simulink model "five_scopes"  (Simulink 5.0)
settings: Solver=ode45  StartTime=0.0  StopTime=10.0  RelTol=1e-3
libraries: xpclib x5

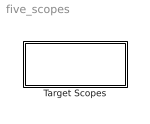
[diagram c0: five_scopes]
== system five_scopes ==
  Target Scopes : Subsystem

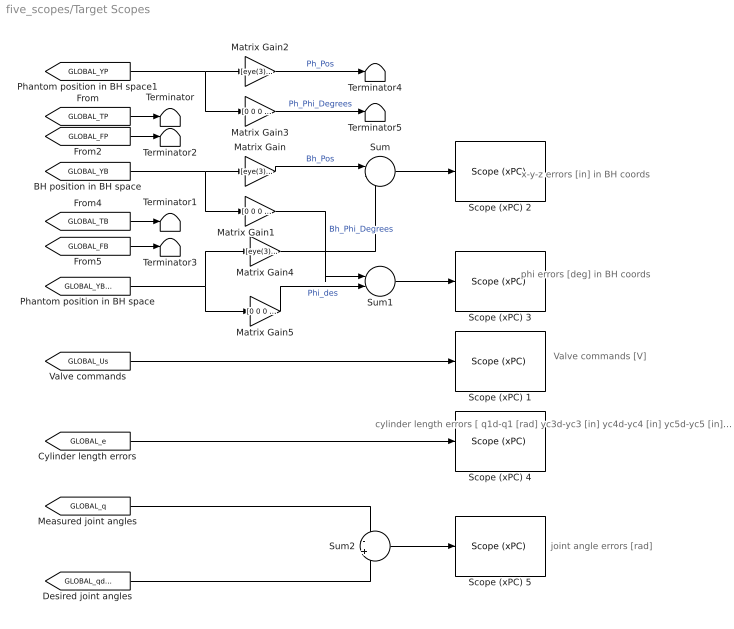
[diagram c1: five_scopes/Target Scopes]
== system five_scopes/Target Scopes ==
  note: x-y-z errors [in] in BH coords
  note: phi errors [deg] in BH coords
  note: Valve commands [V]
  note: cylinder length errors [ q1d-q1 [rad] yc3d-yc3 [in] yc4d-yc4 [in] yc5d-yc5 [in] ]
  note: joint angle errors [rad]
  Matrix Gain : Gain  Gain=[eye(3) zeros(3,1)]  Multiplication=Matrix(K*u)
  Matrix Gain1 : Gain  Gain=[0 0 0 180/pi]  Multiplication=Matrix(K*u)
  Matrix Gain2 : Gain  Gain=[eye(3) zeros(3,1)]  Multiplication=Matrix(K*u)
  Matrix Gain3 : Gain  Gain=[0 0 0 180/pi]  Multiplication=Matrix(K*u)
  Matrix Gain4 : Gain  Gain=[eye(3) zeros(3,1)]  Multiplication=Matrix(K*u)
  Matrix Gain5 : Gain  Gain=[0 0 0 180/pi]  Multiplication=Matrix(K*u)
  Scope (xPC) 1 : xpclib/Misc./Scope (xPC)   scopeno=6  scopetype=Target  viewmode=Graphical redraw  grid=on  ylimits=[0,12]  autostart=on  nosamples=1000  noprepostsamples=0  interleave=1  triggermode=FreeRun  triggersignal=1  triggerlevel=0.0  triggerslope=either  triggerscope=1  triggersample=0
  Scope (xPC) 2 : xpclib/Misc./Scope (xPC)   scopeno=3  scopetype=Target  viewmode=Graphical redraw  grid=on  ylimits=[-10,10]  autostart=off  nosamples=1000  noprepostsamples=0  interleave=1  triggermode=FreeRun  triggersignal=1  triggerlevel=0.0  triggerslope=either  triggerscope=1  triggersample=0
  Scope (xPC) 3 : xpclib/Misc./Scope (xPC)   scopeno=7  scopetype=Target  viewmode=Graphical redraw  grid=on  ylimits=[-10,10]  autostart=off  nosamples=1000  noprepostsamples=0  interleave=1  triggermode=FreeRun  triggersignal=1  triggerlevel=0.0  triggerslope=either  triggerscope=1  triggersample=0
  Scope (xPC) 4 : xpclib/Misc./Scope (xPC)   scopeno=8  scopetype=Target  viewmode=Graphical redraw  grid=on  ylimits=[-5,5]  autostart=on  nosamples=1000  noprepostsamples=0  interleave=1  triggermode=FreeRun  triggersignal=1  triggerlevel=0.0  triggerslope=either  triggerscope=1  triggersample=0
  Scope (xPC) 5 : xpclib/Misc./Scope (xPC)   scopeno=4  scopetype=Target  viewmode=Graphical redraw  grid=on  ylimits=[-.5,.5]  autostart=on  nosamples=1000  noprepostsamples=0  interleave=1  triggermode=FreeRun  triggersignal=1  triggerlevel=0.0  triggerslope=either  triggerscope=1  triggersample=0
  Sum : Sum  Inputs=|-+
  Sum1 : Sum  Inputs=|-+
  Sum2 : Sum  Inputs=-+
  Terminator{,1..5} (6 alike) : Terminator
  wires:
  [GLOBAL_TP] -> Terminator/1
  [GLOBAL_TB] -> Terminator1/1
  [GLOBAL_YB] -> Matrix Gain/1, Matrix Gain1/1
  [GLOBAL_YP] -> Matrix Gain2/1, Matrix Gain3/1
  [GLOBAL_FP] -> Terminator2/1
  [GLOBAL_FB] -> Terminator3/1
  Sum1/1 -> Scope (xPC) 3/1
  Matrix Gain5/1 -> Sum1/2  "Phi_des"
  Matrix Gain1/1 -> Sum1/1  "Bh_Phi_Degrees"
  Sum/1 -> Scope (xPC) 2/1
  Matrix Gain/1 -> Sum/1  "Bh_Pos"
  Matrix Gain4/1 -> Sum/2
  Matrix Gain2/1 -> Terminator4/1  "Ph_Pos"
  Matrix Gain3/1 -> Terminator5/1  "Ph_Phi_Degrees"
  [GLOBAL_Us] -> Scope (xPC) 1/1
  Sum2/1 -> Scope (xPC) 5/1
  [GLOBAL_YB_DES] -> Matrix Gain4/1, Matrix Gain5/1
  [GLOBAL_e] -> Scope (xPC) 4/1
  [GLOBAL_q] -> Sum2/1
  [GLOBAL_qdes] -> Sum2/2
